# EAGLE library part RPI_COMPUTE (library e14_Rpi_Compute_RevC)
Device for a Raspberry PI Compute module. Note that the package is for a DDR2 connector of 'standard' orientation. Example: TE Connectivity P/N: 1565917-4, Newark P/N: 08P0616, Farnell P/N: 2112525 More information is available at http://www.element14.com/community/community/raspberry-pi/raspberry-pi-compute-module
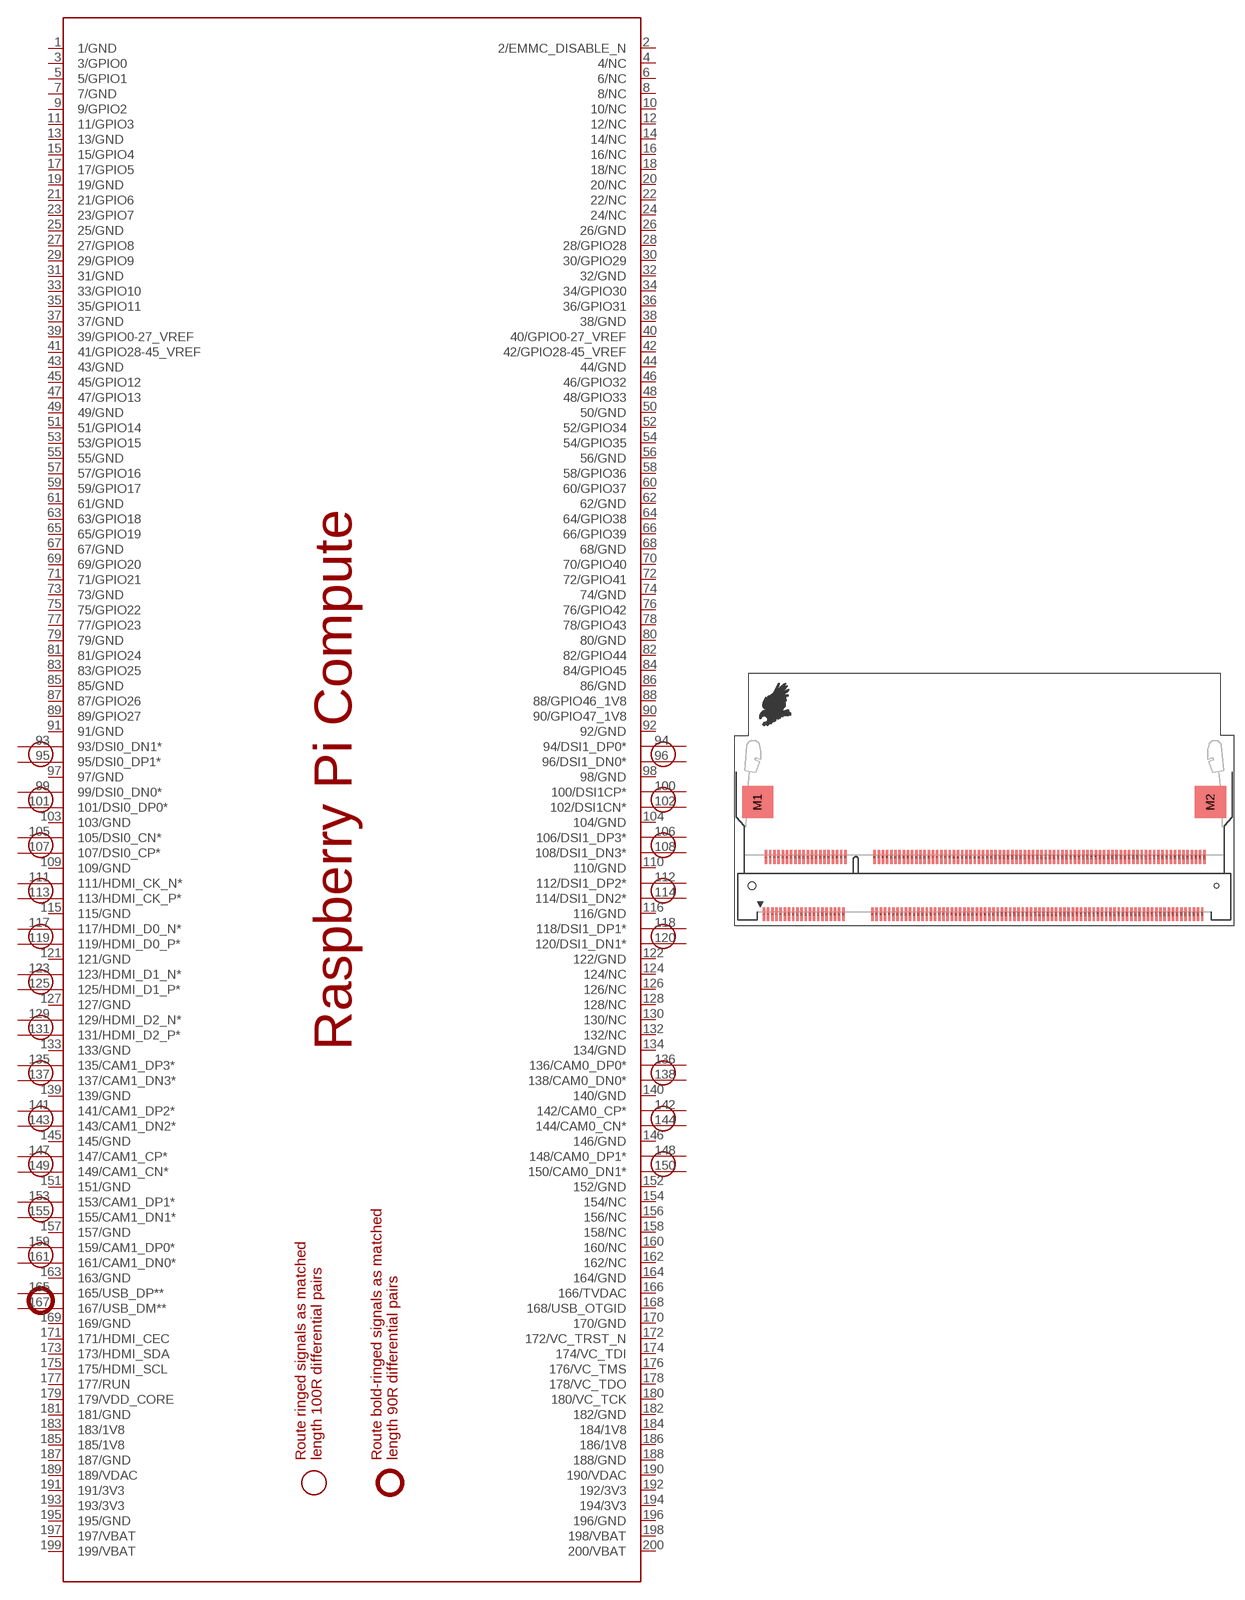
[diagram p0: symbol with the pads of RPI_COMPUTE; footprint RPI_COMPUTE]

Designator prefix PCB

## RPI_COMPUTE  [RPI_COMPUTE]
1  1/GND
2  2/EMMC_DISABLE_N
3  3/GPIO0
4  4/NC
5  5/GPIO1
6  6/NC
7  7/GND
8  8/NC
9  9/GPIO2
10  10/NC
11  11/GPIO3
12  12/NC
13  13/GND
14  14/NC
15  15/GPIO4
16  16/NC
17  17/GPIO5
18  18/NC
19  19/GND
20  20/NC
21  21/GPIO6
22  22/NC
23  23/GPIO7
24  24/NC
25  25/GND
26  26/GND
27  27/GPIO8
28  28/GPIO28
29  29/GPIO9
30  30/GPIO29
31  31/GND
32  32/GND
33  33/GPIO10
34  34/GPIO30
35  35/GPIO11
36  36/GPIO31
37  37/GND
38  38/GND
39  39/GPIO0-27_VREF
40  40/GPIO0-27_VREF
41  41/GPIO28-45_VREF
42  42/GPIO28-45_VREF
43  43/GND
44  44/GND
45  45/GPIO12
46  46/GPIO32
47  47/GPIO13
48  48/GPIO33
49  49/GND
50  50/GND
51  51/GPIO14
52  52/GPIO34
53  53/GPIO15
54  54/GPIO35
55  55/GND
56  56/GND
57  57/GPIO16
58  58/GPIO36
59  59/GPIO17
60  60/GPIO37
61  61/GND
62  62/GND
63  63/GPIO18
64  64/GPIO38
65  65/GPIO19
66  66/GPIO39
67  67/GND
68  68/GND
69  69/GPIO20
70  70/GPIO40
71  71/GPIO21
72  72/GPIO41
73  73/GND
74  74/GND
75  75/GPIO22
76  76/GPIO42
77  77/GPIO23
78  78/GPIO43
79  79/GND
80  80/GND
81  81/GPIO24
82  82/GPIO44
83  83/GPIO25
84  84/GPIO45
85  85/GND
86  86/GND
87  87/GPIO26
88  88/GPIO46_1V8
89  89/GPIO27
90  90/GPIO47_1V8
91  91/GND
92  92/GND
93  93/DSI0_DN1*
94  94/DSI1_DP0*
95  95/DSI0_DP1*
96  96/DSI1_DN0*
97  97/GND
98  98/GND
99  99/DSI0_DN0*
100  100/DSI1CP*
101  101/DSI0_DP0*
102  102/DSI1CN*
103  103/GND
104  104/GND
105  105/DSI0_CN*
106  106/DSI1_DP3*
107  107/DSI0_CP*
108  108/DSI1_DN3*
109  109/GND
110  110/GND
111  111/HDMI_CK_N*
112  112/DSI1_DP2*
113  113/HDMI_CK_P*
114  114/DSI1_DN2*
115  115/GND
116  116/GND
117  117/HDMI_D0_N*
118  118/DSI1_DP1*
119  119/HDMI_D0_P*
120  120/DSI1_DN1*
121  121/GND
122  122/GND
123  123/HDMI_D1_N*
124  124/NC
125  125/HDMI_D1_P*
126  126/NC
127  127/GND
128  128/NC
129  129/HDMI_D2_N*
130  130/NC
131  131/HDMI_D2_P*
132  132/NC
133  133/GND
134  134/GND
135  135/CAM1_DP3*
136  136/CAM0_DP0*
137  137/CAM1_DN3*
138  138/CAM0_DN0*
139  139/GND
140  140/GND
141  141/CAM1_DP2*
142  142/CAM0_CP*
143  143/CAM1_DN2*
144  144/CAM0_CN*
145  145/GND
146  146/GND
147  147/CAM1_CP*
148  148/CAM0_DP1*
149  149/CAM1_CN*
150  150/CAM0_DN1*
151  151/GND
152  152/GND
153  153/CAM1_DP1*
154  154/NC
155  155/CAM1_DN1*
156  156/NC
157  157/GND
158  158/NC
159  159/CAM1_DP0*
160  160/NC
161  161/CAM1_DN0*
162  162/NC
163  163/GND
164  164/GND
165  165/USB_DP**
166  166/TVDAC
167  167/USB_DM**
168  168/USB_OTGID
169  169/GND
170  170/GND
171  171/HDMI_CEC
172  172/VC_TRST_N
173  173/HDMI_SDA
174  174/VC_TDI
175  175/HDMI_SCL
176  176/VC_TMS
177  177/RUN
178  178/VC_TDO
179  179/VDD_CORE
180  180/VC_TCK
181  181/GND
182  182/GND
183  183/1V8
184  184/1V8
185  185/1V8
186  186/1V8
187  187/GND
188  188/GND
189  189/VDAC
190  190/VDAC
191  191/3V3
192  192/3V3
193  193/3V3
194  194/3V3
195  195/GND
196  196/GND
197  197/VBAT
198  198/VBAT
199  199/VBAT
200  200/VBAT

## Footprint RPI_COMPUTE (pad centres in mm)
Package for a DDR2 connector to be used with the Raspberry Pi Compute. Example: TE Connectivity P/N: 1565917-4, Newark P/N: 08P0616, Farnell P/N: 2112525
smd 0.35 x 2: 1 -31.38,-4.1; 2 -31.08,4.1; 3 -30.78,-4.1; 4 -30.48,4.1; 5 -30.18,-4.1; 6 -29.88,4.1; 7 -29.58,-4.1; 8 -29.28,4.1; 9 -28.98,-4.1; 10 -28.68,4.1; 11 -28.38,-4.1; 12 -28.08,4.1; 13 -27.78,-4.1; 14 -27.48,4.1; 15 -27.18,-4.1; 16 -26.88,4.1; 17 -26.58,-4.1; 18 -26.28,4.1; 19 -25.98,-4.1; 20 -25.68,4.1; 21 -25.38,-4.1; 22 -25.08,4.1; 23 -24.78,-4.1; 24 -24.48,4.1; 25 -24.18,-4.1; 26 -23.88,4.1; 27 -23.58,-4.1; 28 -23.28,4.1; 29 -22.98,-4.1; 30 -22.68,4.1; 31 -22.38,-4.1; 32 -22.08,4.1; 33 -21.78,-4.1; 34 -21.48,4.1; 35 -21.18,-4.1; 36 -20.88,4.1; 37 -20.58,-4.1; 38 -20.28,4.1; 39 -19.98,-4.1; 40 -19.68,4.1; 41 -15.78,-4.1; 42 -15.48,4.1; 43 -15.18,-4.1; 44 -14.88,4.1; 45 -14.58,-4.1; 46 -14.28,4.1; 47 -13.98,-4.1; 48 -13.68,4.1; 49 -13.38,-4.1; 50 -13.08,4.1; 51 -12.78,-4.1; 52 -12.48,4.1; 53 -12.18,-4.1; 54 -11.88,4.1; 55 -11.58,-4.1; 56 -11.28,4.1; 57 -10.98,-4.1; 58 -10.68,4.1; 59 -10.38,-4.1; 60 -10.08,4.1; 61 -9.78,-4.1; 62 -9.48,4.1; 63 -9.18,-4.1; 64 -8.88,4.1; 65 -8.58,-4.1; 66 -8.28,4.1; 67 -7.98,-4.1; 68 -7.68,4.1; 69 -7.38,-4.1; 70 -7.08,4.1; 71 -6.78,-4.1; 72 -6.48,4.1; 73 -6.18,-4.1; 74 -5.88,4.1; 75 -5.58,-4.1; 76 -5.28,4.1; 77 -4.98,-4.1; 78 -4.68,4.1; 79 -4.38,-4.1; 80 -4.08,4.1; 81 -3.78,-4.1; 82 -3.48,4.1; 83 -3.18,-4.1; 84 -2.88,4.1; 85 -2.58,-4.1; 86 -2.28,4.1; 87 -1.98,-4.1; 88 -1.68,4.1; 89 -1.38,-4.1; 90 -1.08,4.1; 91 -0.78,-4.1; 92 -0.48,4.1; 93 -0.18,-4.1; 94 0.12,4.1; 95 0.42,-4.1; 96 0.72,4.1; 97 1.02,-4.1; 98 1.32,4.1; 99 1.62,-4.1; 100 1.92,4.1; 101 2.22,-4.1; 102 2.52,4.1; 103 2.82,-4.1; 104 3.12,4.1; 105 3.42,-4.1; 106 3.72,4.1; 107 4.02,-4.1; 108 4.32,4.1; 109 4.62,-4.1; 110 4.92,4.1; 111 5.22,-4.1; 112 5.52,4.1; 113 5.82,-4.1; 114 6.12,4.1; 115 6.42,-4.1; 116 6.72,4.1; 117 7.02,-4.1; 118 7.32,4.1; 119 7.62,-4.1; 120 7.92,4.1; 121 8.22,-4.1; 122 8.52,4.1; 123 8.82,-4.1; 124 9.12,4.1; 125 9.42,-4.1; 126 9.72,4.1; 127 10.02,-4.1; 128 10.32,4.1; 129 10.62,-4.1; 130 10.92,4.1; 131 11.22,-4.1; 132 11.52,4.1; 133 11.82,-4.1; 134 12.12,4.1; 135 12.42,-4.1; 136 12.72,4.1; 137 13.02,-4.1; 138 13.32,4.1; 139 13.62,-4.1; 140 13.92,4.1; 141 14.22,-4.1; 142 14.52,4.1; 143 14.82,-4.1; 144 15.12,4.1; 145 15.42,-4.1; 146 15.72,4.1; 147 16.02,-4.1; 148 16.32,4.1; 149 16.62,-4.1; 150 16.92,4.1; 151 17.22,-4.1; 152 17.52,4.1; 153 17.82,-4.1; 154 18.12,4.1; 155 18.42,-4.1; 156 18.72,4.1; 157 19.02,-4.1; 158 19.32,4.1; 159 19.62,-4.1; 160 19.92,4.1; 161 20.22,-4.1; 162 20.52,4.1; 163 20.82,-4.1; 164 21.12,4.1; 165 21.42,-4.1; 166 21.72,4.1; 167 22.02,-4.1; 168 22.32,4.1; 169 22.62,-4.1; 170 22.92,4.1; 171 23.22,-4.1; 172 23.52,4.1; 173 23.82,-4.1; 174 24.12,4.1; 175 24.42,-4.1; 176 24.72,4.1; 177 25.02,-4.1; 178 25.32,4.1; 179 25.62,-4.1; 180 25.92,4.1; 181 26.22,-4.1; 182 26.52,4.1; 183 26.82,-4.1; 184 27.12,4.1; 185 27.42,-4.1; 186 27.72,4.1; 187 28.02,-4.1; 188 28.32,4.1; 189 28.62,-4.1; 190 28.92,4.1; 191 29.22,-4.1; 192 29.52,4.1; 193 29.82,-4.1; 194 30.12,4.1; 195 30.42,-4.1; 196 30.72,4.1; 197 31.02,-4.1; 198 31.32,4.1; 199 31.62,-4.1; 200 31.92,4.1
smd 4.5 x 4.6: M1 -32.28,12; M2 32.82,12
hole 1.1 at -33.13,0
hole 0.6 at 33.67,0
